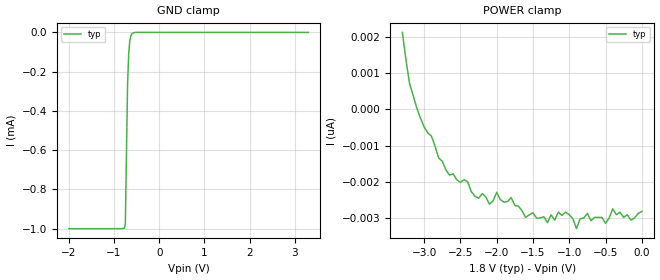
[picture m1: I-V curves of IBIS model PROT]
| Texas Instruments Incorporated
| USB Type-C Port Protector: Short-to-VBUS Overvoltage and IEC ESD Protection
| Marketing part#   Voltage Range   Package-type   #pins/pkg drawing
| TPD8S300RUK   2.7V - 3.6V   WQFN   20-pin RUK
[IBIS Ver]   4.1
[File name]   tpd8s300.ibs
[File Rev]   1.0
[Date]   11/11/2016
[Source]   Model built from from bench measurements at:
   Texas Instruments Incorporated.
   Analog-eLab, HPA
   12500 TI Blvd
   Dallas, TX -75243
   For Support e-mail: elab_ibis@list.ti.com
[Notes]   Revision History
   Rev 1.0: 11/11/2016
   c_comp values not available. Nominal values put in place to avoid errors
[Disclaimer]  This model is designed as an aid for customers of Texas Instruments
 TI and its licensors and suppliers make no warranties, either expressed
 or implied, with respect to this  model, including the warranties of
 merchantability or fitness for a particular purpose.
 The model is provided solely on an "as is" basis. The entire risk as to
 its quality and performance is with the customer.
[Copyright] (C)Copyright 2016 Texas Instruments Incorporated.
   All rights reserved.
[Component]   TPD8S300RUK
[Manufacturer]  Texas Instruments Incorporated
[Package]   |20-pin BGA package
|   typ   min   max
R_pkg   0.005   0.005   0.005
L_pkg   0.20nH   0.2nH   0.2nH
C_pkg   0.6pF   0.6pF   0.6pF
[Pin]   signal_name   model_name   R_pin   L_pin   C_pin
1   C_SBU1   NC   0.005   0.2nH   0.6pF
2   C_SBU1   NC   0.005   0.2nH   0.6pF
3   VBIAS   NC   0.005   0.2nH   0.6pF
4   C_CC1   NC   0.005   0.2nH   0.6pF
5   C_CC2   NC   0.005   0.2nH   0.6pF
6   RPD_G2   NC   0.005   0.2nH   0.6pF
7   RPD_G1   NC   0.005   0.2nH   0.6pF
8   GND   GND   0.005   0.2nH   0.6pF
9   FLTB   NC   0.005   0.2nH   0.6pF
10   VPWR   POWER   0.005   0.2nH   0.6pF
11   CC2   NC   0.005   0.2nH   0.6pF
12   CC1   NC   0.005   0.2nH   0.6pF
13   GND   GND   0.005   0.2nH   0.6pF
14   SBU2   NC   0.005   0.2nH   0.6pF
15   SBU1   NC   0.005   0.2nH   0.6pF
16   D4   PROT   0.005   0.2nH   0.6pF
17   D3   PROT   0.005   0.2nH   0.6pF
18   GND   GND   0.005   0.2nH   0.6pF
19   D2   PROT   0.005   0.2nH   0.6pF
20   D1   PROT   0.005   0.2nH   0.6pF
| Models and submodels in the file (1): PROT (Input)
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|   Model sdascl
[Model]   PROT
Model_type   Input
Vinl = 0.4
Vinh = 1.2
|   typ   min   max
C_comp   0.06p   0.05p   0.07p
[Voltage Range]   3.3   2.7   3.6
[Temperature Range]   27   125   -40
[Power Clamp Reference]   1.8   1.62   1.98
[GND Clamp Reference]   0   0   0
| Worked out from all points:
|   GND clamp passes 1 mA (typ) near -0.90 V on its own axis
[GND Clamp]
|   Voltage   I(typ)   I(min)   I(max)
-2V       -1mA       NA         NA
-775mV    -998.2uA   NA         NA
-750mV    -978.2uA   NA         NA
-725mV    -614.7uA   NA         NA
-700mV    -261.2uA   NA         NA
-675mV    -105.1uA   NA         NA
-650mV    -41.17uA   NA         NA
-625mV    -15.86uA   NA         NA
-600mV    -6.087uA   NA         NA
-475mV    -52.56nA   NA         NA
3.3V      -2.815nA   NA         NA
[POWER Clamp]
|   Voltage   NA  I(typ)   I(min)   I(max)
-3.3V     2.119nA    NA         NA
-3.2V     698.7pA    NA         NA
-3V       -484.8pA   NA         NA
-2.65V    -1.814nA   NA         NA
-2.3V     -2.397nA   NA         NA
-2.1V     -2.615nA   NA         NA
-2V       -2.287nA   NA         NA
-1.3V     -3.125nA   NA         NA
-1.05V    -2.834nA   NA         NA
-900mV    -3.289nA   NA         NA
-750mV    -2.87nA    NA         NA
0V        -2.815nA   NA         NA
